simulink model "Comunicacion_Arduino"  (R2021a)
settings: Solver=VariableStepAuto  StartTime=0.0  StopTime=60  RelTol=1e-3
undefined symbols (not defined in the file or in its folder): LF
libraries: instrumentseriallib x3

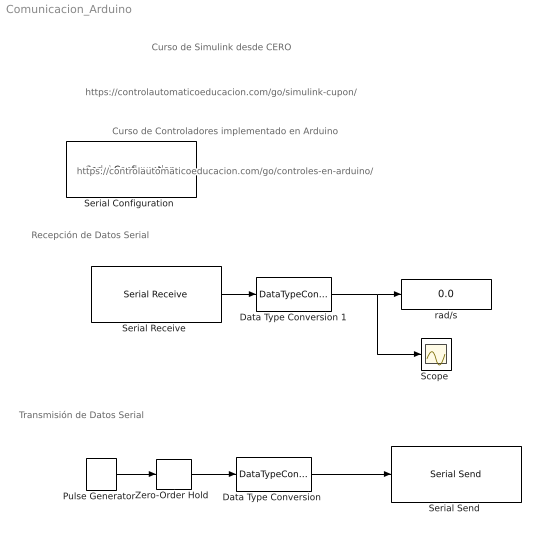
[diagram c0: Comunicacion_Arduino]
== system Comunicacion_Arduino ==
  note: Transmisión de Datos Serial
  note: Recepción de Datos Serial
  note: Curso de Simulink desde CERO
  note: https://controlautomaticoeducacion.com/go/simulink-cupon/
  note: https://controlautomaticoeducacion.com/go/controles-en-arduino/
  note: Curso de Controladores implementado en Arduino
  "Data Type Conversion " : DataTypeConversion  OutDataTypeStr=single
  Data Type Conversion 1 : DataTypeConversion  OutDataTypeStr=double
  "Pulse Generator " : DiscretePulseGenerator  PulseType=Time based  Amplitude=5  Period=4  PulseWidth=50
  "Scope " : Scope
  "Serial Configuration " : instrumentseriallib/Serial Configuration  Priority=-200000  Port=COM1  ComPort=COM1  BaudRate=9600  DataBits=8  Parity=none  StopBits=1  ByteOrder=little-endian  FlowControl=none  Timeout=10  SimulateUsing=Interpreted execution  BlockInModel=on
  "Serial Receive " : instrumentseriallib/Serial Receive  Priority=1  Port=COM1  ComPort=COM1  DataType=single  SaveDataType=uint8  ToggleHeader=on  Header='V'  ToggleTerminator=on  Terminator=LF ('\n')  CustomTerminator=[]  ToggleDataSize=on  DataSize=[1 1]  EnableBlockingMode=on  ActionDataUnavailable=Output last received value  ActionWhenDataUnavailable=Output last received value  CustomValue=0  SampleTime=0.05  SimulateUsing=Interpreted execution  BlockInModel=on
  "Serial Send " : instrumentseriallib/Serial Send  Priority=1  Port=COM1  ComPort=COM1  Header=[]  Terminator=<none>  CustomTerminator=[]  EnableBlockingMode=on  SimulateUsing=Interpreted execution  BlockInModel=on
  "Zero-Order Hold " : ZeroOrderHold  SampleTime=0.05
  rad/s : Display
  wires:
  "Pulse Generator "/1 -> "Zero-Order Hold "/1
  "Zero-Order Hold "/1 -> "Data Type Conversion "/1
  "Data Type Conversion "/1 -> "Serial Send "/1
  "Serial Receive "/1 -> Data Type Conversion 1/1
  Data Type Conversion 1/1 -> "Scope "/1, rad/s/1
